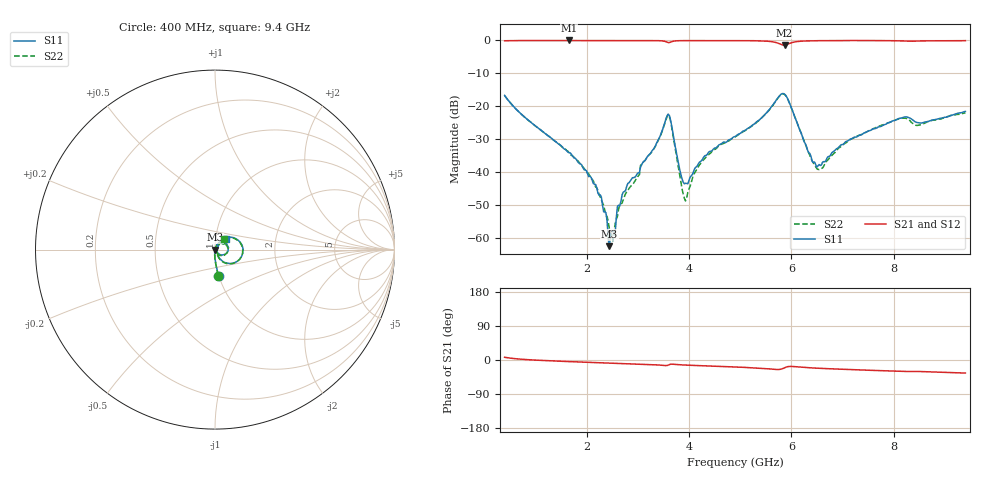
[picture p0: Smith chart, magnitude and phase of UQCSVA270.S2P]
!  Part Number  UQCSVA270  Mounting Orientation: Horizontal
!  Description: Ultra Low ESR Microwave capacitors
!  Application: Coupling, Bypass, Tuning, DC Block
!  Filters, Matching
# GHZ S DB R 50
! Freq  |S11|  S11 Ph  |S21|  S21 Ph  |S12|  S12 Ph  |S22|  S22 Ph
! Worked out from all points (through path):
!   401 points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, 400 MHz to 9.4 GHz, reference 50 ohm
!   highest |S21| = 0.00 dB at 1.66 GHz (marker M1); lowest = -1.4 dB at 5.868 GHz (marker M2)
!   group delay of S21, straight-line fit = 11 ps
!   lowest |S11| = -62.5 dB at 2.448 GHz (marker M3), VSWR 1.00, Z = 50 - j0.0636 ohm
!   |S11| at or under -10 dB: start of sweep to end of sweep
!   |S22| runs from -60.9 to -16.2 dB; largest |S21 - S12| = 0.0031
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0.4  -16.69 -82.2  -0.11 7.2  -0.12 7.1  -16.72 -82.4
1.66  -34.10 -93.4  0.00 -4.2  -0.01 -4.3  -34.08 -96.0
1.908  -37.84 -99.1  0.00 -5.5  -0.02 -5.5  -38.13 -94.3
2.245  -46.95 -100.2  0.00 -7.1  -0.01 -7.1  -46.82 -87.9
2.448  -62.46 -122.3  -0.01 -8.0  -0.01 -8.1  -57.36 -46.5
2.515  -57.92 128.2  -0.01 -8.3  -0.01 -8.4  -60.86 6.3
2.74  -45.88 89.2  0.00 -9.4  -0.02 -9.4  -47.41 63.2
3.415  -29.77 64.3  -0.07 -13.3  -0.08 -13.3  -29.87 60.6
3.618  -22.77 -8.8  -0.64 -12.2  -0.65 -12.2  -23.08 -15.2
3.843  -40.71 -33.7  -0.06 -12.8  -0.07 -12.8  -42.97 -50.2
3.933  -43.37 7.7  -0.05 -13.4  -0.06 -13.4  -48.72 10.4
4.27  -35.94 63.8  -0.03 -15.2  -0.04 -15.2  -36.49 68.9
4.9  -29.17 61.8  -0.04 -18.4  -0.05 -18.4  -29.29 63.9
5.665  -19.06 38.1  -0.49 -24.6  -0.50 -24.5  -19.12 37.2
5.868  -16.31 -14.3  -1.41 -20.4  -1.42 -20.3  -16.37 -15.8
6.408  -36.67 -39.3  -0.10 -21.0  -0.11 -20.9  -36.65 -45.2
6.565  -37.98 4.4  -0.07 -22.1  -0.07 -22.0  -39.06 4.8
7.15  -29.99 49.7  -0.02 -25.1  -0.02 -25.1  -30.08 52.3
7.915  -24.91 52.0  -0.07 -28.9  -0.08 -28.9  -24.89 50.4
8.208  -23.24 42.2  -0.18 -30.2  -0.19 -30.2  -23.62 38.9
8.478  -24.97 35.9  -0.17 -30.3  -0.17 -30.2  -25.75 43.2
9.4  -21.56 45.4  -0.06 -34.5  -0.07 -34.5  -21.97 48.9
